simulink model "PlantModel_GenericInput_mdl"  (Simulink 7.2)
settings: Solver=ode45  StartTime=0.0  StopTime=10  RelTol=1e-3
InitFcn:
  | s = tf('s');
  | G_plant = (101*s + 808)/(s^3 + 6*s^2 + 109*s + 404);
  | Gd_plant = tf(c2d(G_plant,Ts,'zoh'))
  | [B_plant,A_plant] = tfdata(Gd_plant,'v');
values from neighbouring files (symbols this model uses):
  Ts = 0.01    [Esercitazione03.m]
undefined symbols (not defined in the file or in its folder): A_plant, polyval
libraries: simulink x1, cstblocks x1

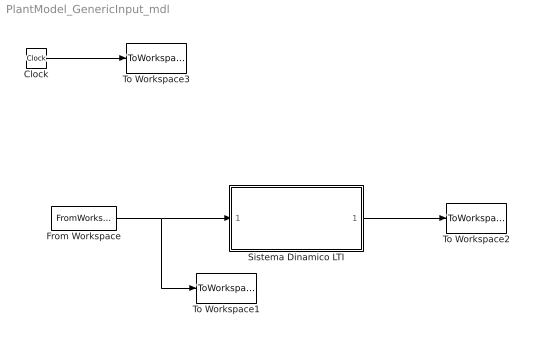
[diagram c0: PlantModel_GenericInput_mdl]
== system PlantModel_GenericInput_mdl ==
  Clock : Clock
  From Workspace : FromWorkspace  VariableName=[timed ui]  SampleTime=0
  Sistema Dinamico LTI : Subsystem
  To Workspace1 : ToWorkspace  VariableName=u  SampleTime=Ts  SaveFormat=Array
  To Workspace2 : ToWorkspace  VariableName=y  SampleTime=Ts  SaveFormat=Array
  To Workspace3 : ToWorkspace  VariableName=time  SampleTime=-1  SaveFormat=Array
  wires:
  From Workspace/1 -> To Workspace1/1, Sistema Dinamico LTI/1(u)
  Sistema Dinamico LTI/1(y) -> To Workspace2/1
  Clock/1 -> To Workspace3/1

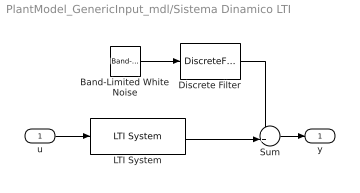
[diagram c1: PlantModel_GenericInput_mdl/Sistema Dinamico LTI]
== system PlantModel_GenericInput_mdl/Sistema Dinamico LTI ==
  u : Inport
  Band-Limited White Noise : simulink/Sources/Band-Limited White Noise  SystemSampleTime=-1  Cov=0.0001  Ts=Ts  seed=[23341]
  Discrete Filter : DiscreteFilter  Numerator=polyval(A_plant,1)*[1]  Denominator=A_plant  SampleTime=Ts
  LTI System : cstblocks/LTI System  SystemSampleTime=-1  sys=Gd_plant  IC=[]
  Sum : Sum  Inputs=++|  OutDataType=sfix(16)  OutScaling=2^0
  y : Outport
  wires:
  LTI System/1 -> Sum/2
  u/1 -> LTI System/1
  Sum/1 -> y/1
  Band-Limited White Noise/1 -> Discrete Filter/1
  Discrete Filter/1 -> Sum/1
